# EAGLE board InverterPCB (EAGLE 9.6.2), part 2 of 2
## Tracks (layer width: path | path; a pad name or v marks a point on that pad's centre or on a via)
ADC1_IN8
  Route2 0.25: C57.2 63.3,58.52 | J2.34 65.97,61.19 63.3,58.52 | R124.1 62.62,59.21 63.3,58.52
ADC1_IN10
  Route2 0.25: J2.38 65.44,66.27 C39.2 62.34,63.81 R61.1
ADC1_IN11
  Route15 0.25: J2.36 65.87,66.01 56.33,66.01 C48.2 52.84,69.03 R109.1
ADC2_IN9
  Route2 0.25: J1.24 129.14,48.51 C60.2 122.55,48.51 R129.1
ADC2_IN12
  Route15 0.25: J2.35 71.97,65.01 85.73,65.01 C42.2 88.64,63.3 R99.1
ADC2_IN13
  Route2 0.25: J2.37 73.86,66.27 C51.2 77.61,63.33 R114.1
ADC3_IN0
  Route2 0.25: R104.1 60.71,46.14 63.27,48.7 | J2.28 63.69,49.11 63.27,48.7 | C45.2 63.27,48.7
ADC3_IN1
  Route15 0.25: J2.30 67.05,55.01 54.92,55.01 C54.2 52.53,56.56 R119.1
CURENT_MEAS_DC_LINK
  Top 0.25: IC26.13 IC26.14 | R125.2 230.21,54.75 J23.1
  Route15 0.25: J23.1 232.47,57.01 247.79,57.01 256.15,65.37 IC26.14
CURENT_MEAS_PHASE_1
  Top 0.25: IC26.2 IC26.1
  Top 0.254: IC20.6 250.79,80 250.79,73.01 252.04,71.76 259.04,71.76 260.28,70.52 263.74,70.52 IC26.2
  Bottom 0.254: IC21.7 236.87,84.93 237.79,84.01 246.78,84.01 IC20.6
CURENT_MEAS_PHASE_2
  Top 0.25: IC26.6 IC26.7
  Bottom 0.254: IC26.6 260.84,80.71 259.55,79.42 254.2,79.42 252.29,77.51 IC20.4 245.08,77.51 243.81,78.78 237.02,78.78 235.95,79.85 IC21.5
CURENT_MEAS_PHASE_3
  Top 0.25: IC26.9 IC26.8
  Top 0.254: IC26.8 252.38,87.01 242.46,87.01 IC20.8
  Bottom 0.254: IC20.8 240.58,87.22 239.79,88.01 229.79,88.01 228.79,87.01 228.79,84.01 227.17,82.39 IC21.9
CURRENT_MEAS_PHASE_1_GRID
  Top 0.25: J15.1 253.39,55.17 R105.2
  Bottom 0.2: IC4.1 IC4.2
  Bottom 0.25: R105.2 266.38,61.01 295.51,61.01 IC4.1
CURRENT_MEAS_PHASE_2_GRID
  Top 0.25: J17.1 281.7,55.4 R110.2
  Bottom 0.2: IC4.7 302.66,83.2 302.66,80.76
  Bottom 0.25: J17.1 279.41,60.01 300.79,60.01 304.79,64.01 304.79,79.01 303.04,80.76 302.66,80.76 IC4.6
CURRENT_MEAS_PHASE_3_GRID
  Top 0.25: R115.2 296.79,55.28 J19.1
  Route15 0.25: J19.1 296.74,78.96 296.79,79.01 295.04,80.76 IC4.9 IC4.8
DC_LINK_NEGATIVE_OUT
  Top 0.25: J5.1 85.23,182.66 VR7.1
  Top 1: R36.2 134.95,157.49 D6.A 135.49,166.94 Q2.S | R50.2 D10.A | D10.A | R56.2 274.83,156.03 D13.A 275.34,165.87 Q6.S | Q4.S 204.98,180.14 D10.A
  Bottom 0.25: J5.1 79.93,196.87 79.79,197.01
  Bottom 1: C20.2 123.95,170.01 131.34,170.01 D6.A | C23.2 196.57,172.01 201.79,172.01 204.97,168.83 D10.A | C27.2 265.3,171.01 270.79,171.01 274.83,166.97 D13.A
  Bottom 3: 47.9,187.42 48.5,188.01 55.79,188.01 64.79,197.01 79.79,197.01 128.79,197.01 | 128.79,197.01 135.79,190.01 135.79,180.72 Q2.S | 128.79,197.01 198.79,197.01 | 198.79,197.01 205.79,190.01 205.79,180.95 Q4.S | 198.79,197.01 268.79,197.01 275.34,190.46 275.34,185.01 Q6.S
  Bottom 4: X3.1 19.9,187.42 D2.A | D2.A D3.A 40.27,187.42 | X3.2 14.9,187.42 D2.A | 40.27,187.42 C73.- | C28.2 47.9,187.42 40.27,187.42
DC_LINK_POSITIVE
  Top 0.254: D3.C D2.C 15.74,196.06 X2.2
  Top 4: X2.1 15.8,196.01 | 15.8,196.01 C73.+ 54.13,196.01 C28.1 | X2.2 15.8,196.01
  pour Top: 63.82,183.1 63.82,193.04 57.16,199.7 38.7,199.7 37.74,198.74 37.74,193.05 38.47,192.32 57.53,192.32 57.62,192.41 60.66,189.37 60.66,183.42 60.98,183.1
DC_LINK_POSITIVE_OUT
  Top 0.25: 67.4,187.01 89.34,187.01 R38.2 97.71,185.31 Q1.D
  Top 0.254: 67.4,187.01 66.26,187.01 66.03,186.78 U11.1
  Top 1: Q1.D 103.03,179.99 D4.C | Q3.D 172.79,166.69 D9.C | Q5.D 242.75,165.4 D12.C
  Bottom 1: Q1.D 107.01,176.01 111.54,176.01 R152.1 | Q3.D 177.17,176.01 181.74,176.01 R154.1 | Q5.D 247.31,175.01 250.34,175.01 R155.1
  pour Top: 64.51,184.13 64.48,185.24 64.48,188.13 75.64,199.29 237.2,199.29 244.96,191.53 244.96,176.06 243.86,174.96 241.31,174.96 239.92,176.35 239.92,190.4 236.08,194.24 181.39,194.24 174.82,187.67 174.82,176.86 173.74,175.78 171.64,175.78 170.56,176.86 170.56,187.74 163.81,194.49 108.8,194.57 105.13,190.9 105.13,190.1 105.07,190.04 105.07,176.91 104.65,176.49 100.06,176.49 99.29,177.26 99.29,190.82 95.62,194.49 77.92,194.49 66.33,182.9
DIGITAL_PROTECTION
  Top 0.25: R30.2 R39.1
  Route15 0.25: R39.1 114.87,53.01 122.65,53.01 123.58,52.07 129.59,52.07 129.65,52.01 130.79,52.01 131.7,51.1 J1.25
ENABLE_PWM  (via drill 0.35)
  Top 0.25: T1.3 144.62,58.05 | 144.62,58.05 T12.3 T11.3 160.52,58.05 T10.3 | R85.2 141.79,52.15 141.79,57.01 142.83,58.05 144.62,58.05 | IC22.10 163.95,92.17 165.79,94.01 190.79,94.01 193.43,91.37 IC25.10 | R30.1 v112.79,70.01
  Route2 0.25: IC22.2 156.33,80.55 155.79,80.01 150.79,80.01 144.5,73.72 v144.5,68.01 T1.3
  Route15 0.25: v112.79,70.01 112.79,76.01 113.79,77.01 v120.79,77.01
  Bottom 0.25: IC22.10 163.95,85.01 | 163.95,85.01 IC22.5 | IC22.2 158.98,85.01 163.95,85.01 | IC25.10 193.43,85.01 | 193.43,85.01 IC25.5 | IC25.2 188.26,85.01 193.43,85.01 | v120.79,77.01 135.5,77.01 v144.5,68.01
GPIO_OUTPUT
  Route15 0.254: IC14.15 136.71,43.39 135.47,44.63 130.48,44.63 J1.22
HIGHSIDE_3V  (via drill 0.35)
  Top 0.25: IC17.4 392.44,70.01 400.79,70.01 401.74,69.06 402.51,69.06 C84.1 402.6,68.97 402.6,63.82 401.79,63.01 400.47,63.01 | 400.47,63.01 383.79,63.01 | 383.79,63.01 365.82,63.01 | 365.82,63.01 346.81,63.01 | 346.81,63.01 R40.2 | R26.2 365.82,63.01 | R15.2 381.8,65 383.79,63.01 | R3.2 400.47,63.01 | 346.81,63.01 341.79,63.01 340.76,64.04 C5.1 338.62,69.18 337.79,70.01 329.79,70.01 328.56,68.78 IC19.4 | C85.1 372.76,74 363.19,74 363.18,74.01 362.63,74.01 IC18.11
  Top 1: IC2.2 37.43,152.83 R69.1
  Route15 0.25: R26.2 362.42,66.41 362.42,74.22 IC18.11
  Route15 1: C2.1 76.49,129.01 141.79,129.01 141.79,128.01 142.79,127.01 v144.79,127.01 | v155.79,127.01 157.79,129.01 213.79,129.01 v215.79,127.01 | v226.79,127.01 228.79,129.01 283.79,129.01 v285.79,127.01 | v303.79,127.01 305.79,129.01 328.79,129.01 338.79,119.01 338.79,71.16 C5.1
  Bottom 0.25: VR1.3 328.56,60.87 IC19.4
  Bottom 1: C2.1 50.12,155.38 50.12,155.89 48.1,157.91 R69.1 | v144.79,127.01 v155.79,127.01 | v215.79,127.01 v226.79,127.01 | v285.79,127.01 v303.79,127.01
HIGHSIDE_5V
  Top 1: C83.1 43.78,141.4 IC5.3 | OK1.8 103.61,128.6 R43.1 96.12,136.09 R42.1 96.16,137.52 C11.1 | C19.1 R52.1 164.94,135.45 R53.1 172.61,127.79 OK2.8 | C24.1 234.64,139.6 R58.1 237.18,132.12 R59.1 242.27,125.76 OK3.8
  Bottom 1: C83.1 93.46,140.13 R42.1 97.58,136.01 164.79,136.01 164.94,136.16 R52.1 167.15,134.66 R58.1
HIGHSIDE_15V_VB  (via drill 0.35)
  Top 1: C15.1 106.28,148.74 U4.8 | D5.C 127.99,146.01 v111.79,146.01
  Bottom 1: v111.79,146.01 108.88,146.01 U4.8
HIGHSIDE_15V_VB1  (via drill 0.35)
  Top 1: C13.1 36.19,127.4 IC9.3 | U4.5 114.92,147.58 C14.1 120.75,147.58 R153.1 | R156.1 189.53,146.73 C21.1 183.91,146.73 U6.5 | R157.1 259.03,144.76 C25.1 253.62,144.76 U7.5
  Route2 1: C13.1 54.56,137.01 v84.79,137.01
  Route15 1: v84.79,137.01 91.79,144.01 112.79,144.01 116.36,147.58 C14.1
  Bottom 1: R153.1 134.56,149.78 139.79,155.01 180.79,155.01 182.8,153 U6.5 | R156.1 195.98,149.2 198.79,152.01 250.79,152.01 252.43,150.37 U7.5
HIGHSIDE_-3V  (via drill 0.35)
  Top 0.25: C84.2 401.9,74.12 400.79,73.01 392.45,73.01 IC17.11 | C85.2 370.58,69.22 369.79,70.01 363.06,70.01 IC18.4
  Top 1: IC3.3 38.7,171.88 R67.2 52.67,171.88 C3.2
  Route2 0.25: C5.2 339.51,73.01 v332.79,73.01
  Route15 0.2: 361.04,68.76 IC18.4
  Route15 0.25: C5.2 350.54,74.26 354.79,70.01 359.79,70.01 360.93,68.88 361.04,68.76 | v332.79,73.01 331.29,73.01 IC19.11
  Route15 1: C3.2 60.79,163.76 60.79,151.01 80.79,131.01 v144.79,131.01 | v157.79,131.01 v215.79,131.01
  Bottom 0.25: C85.2 375.25,71.41 388.19,71.41 390.14,73.36 IC17.11
  Bottom 1: v144.79,131.01 v157.79,131.01 | C5.2 340.76,119.04 327.04,132.76 235.54,132.76 233.79,131.01 v215.79,131.01
HIGHSIDE_GND  (via drill 0.35)
  Top 1: X1.2 15.12,168.59 D1.A 25.48,168.59 C4.2 30.53,168.07 31.8,166.8 IC3.2 | C82.2 28.54,138.86 IC5.2 41.24,138.86 C83.2 | C12.2 29.84,127.46 32.41,124.89 IC9.2 42.38,124.89 C13.2 | C14.2 117.63,143.37 112.95,143.37 111.29,141.72 U4.3 111.29,141.67 108.95,144.01 99,144.01 C11.2 | C21.2 186.43,142.43 181.93,142.43 180.26,140.76 U6.3 180.26,140.78 178.03,143.01 168.79,143.01 C19.2 | C24.2 238.82,140.53 248.28,140.53 249.89,138.93 U7.3 249.89,138.87 251.61,140.59 255.96,140.59 C25.2
  Route2 1: v342.79,88.29 327.07,88.29 323.48,84.7 IC19.13 IC19.12
  Bottom 1: C4.2 29.59,164.48 29.59,144.99 C82.2 | C13.2 49.19,126.56 49.19,131.91 46.05,135.05 C83.2 41.79,138.31 41.79,142.01 43.79,144.01 93.32,144.01 C11.2 | C14.2 120.28,142.5 121.79,144.01 162.1,144.01 C19.2 | C21.2 189.96,141.65 192.39,144.08 234.05,144.08 C24.2 | C25.2 259.37,142.19 320.84,142.19 342.79,120.24 v342.79,88.29
HIGHSIDE_LOW_VOLTAGE_INPUT
  Top 1: X1.1 19.09,161.76 D1.C 24.09,156.77 C1.1 27.3,155.37 IC2.3 | C82.1 IC5.1 | C12.1 36.13,122.38 IC9.1
  Bottom 1: IC2.3 36.14,155.35 32.91,155.35 31.89,154.33 31.89,137.43 33,136.32 | IC5.1 33,136.32 | 33,136.32 31.91,135.23 31.91,124.04 33.63,122.32 36.13,122.32 IC9.1
HIGHSIDE_SPLIT_GND  (via drill 0.35)
  Top 0.2: U1.4 391.97,50.89 378.03,50.89 376.35,52.57
  Top 0.25: U1.4 393.64,58.86 396.79,62.01 403.79,62.01 404.79,63.01 404.79,75.01 402.79,77.01 394.36,77.01 IC17.10 | v371.79,61.01 376.35,56.45 U2.4 376.35,52.57 374.79,51.01 360.44,51.01 | U3.4 360.44,51.01 | 360.44,51.01 341.72,51.01 U5.4 340.11,52.69 336.79,56.01 336.79,63.01 334.79,65.01 327.79,65.01 326.02,66.79 IC19.3 | R12.2 397,154.01 388.62,154.01 R17.2
  Top 1: VR3.2 51.4,166.8 53.94,164.26 C3.1 C2.2 51.4,155.37 | 51.4,155.37 VR2.2 | C4.1 29.01,162.99 32.19,159.81 46.96,159.81 51.4,155.37
  Route2 0.25: v371.79,61.01 370.55,61.01 IC18.5 | v381.79,88.01 381.79,84.01 386.79,79.01 388.99,79.01 IC17.10
  Route2 1: C2.2 71.43,155.37 97.79,129.01 v144.79,129.01 114.54,129.01 OK1.5 | IC19.10 331.1,73.2 IC19.3
  Bottom 0.25: R17.2 383.79,153.15 383.79,118.01 | R28.2 372.75,121.05 374.79,119.01 382.79,119.01 383.79,118.01 | 383.79,118.01 383.79,99.01 381.79,97.01 v381.79,88.01
  Bottom 1: C4.1 23.19,160.18 23.19,154.4 C1.2 | v144.79,129.01 181.79,129.01 | 181.79,129.01 251.79,129.01 | OK2.5 180.23,127.45 181.79,129.01 | OK3.5 249.89,127.11 251.79,129.01 | IC19.10 331.1,78.31 331.79,79.01 335.79,79.01 338.79,82.01 338.79,117.43 327.21,129.01 251.79,129.01
HIGHSIDE_VOFFSET  (via drill 0.35)
  Top 0.2: 358.5,70.58 375.75,70.58 v375.77,70.6
  Top 0.25: C18.1 330.65,56.74 VR1.2 320.47,56.74 J3.2 | IC18.3 358.5,70.58 IC18.12
  Bottom 0.2: IC17.5 392.68,68.73 390.81,70.6 v375.77,70.6
  Bottom 0.25: C18.1 349.77,59.25 IC18.3
LACH_RESET  (via drill 0.35)
  Top 0.25: R81.2 153.59,24.09 SW1.P$2 | IC14.6 173.51,52.25 168.43,52.25 IC14.12 169.76,48.44 | IC14.4 171.07,48.47 171.03,48.44 169.76,48.44 | IC14.14 169.7,48.44 169.76,48.44
  Route2 0.25: R81.2 155.89,24.11 158.79,27.01 v158.79,34.01
  Route15 0.25: v158.79,34.01 161.79,37.01 168.79,37.01 170.79,39.01 170.79,44.01 168.87,45.93 IC14.14
LOWSIDE_3.3V  (via drill 0.35)
  Top 0.25: IC16.4 215.79,24.75 215.79,32.25 C7.1 | IC26.4 263.68,75.63 261.79,77.51 261.79,86.62 C87.1 | C6.1 322.04,34.96 322.04,27.1 324.34,24.8 IC7.4 | IC1.4 214.79,44.44 v214.79,44.01 | v225.79,61.01 258.79,61.01 | v312.79,42.01 310.79,44.01 310.79,69.01 304.12,75.68 IC4.4 | C29.2 295.96,170.62 U10.8 | C74.2 330.35,170.52 U12.8 | C75.2 344.58,134.71 U13.8 | C76.2 359.15,100.37 U14.8 | C10.2 223.76,170.49 U9.8 | C8.2 152.75,171.18 U8.8 | U11.8 66.03,176.25 C33.2 65.79,174.5 65.79,97.93 C32.1
  Top 0.254: 258.79,61.01 263.79,61.01 266.79,64.01 266.79,74.01 265.18,75.62 263.78,75.62 IC26.4
  Top 1: IC15.2 39.97,93.7 R64.1 56.48,88.62 C32.1
  Route2 1: C32.1 72.87,105.01 v153.79,105.01
  Route15 0.25: v214.79,44.01 214.79,35.98 C7.1 | C86.1 221.11,60.34 221.79,61.01 v225.79,61.01 | C6.1 314.99,42.01 v312.79,42.01 | C87.1 262.47,99.33 256.79,105.01 | C8.2 153.24,105.56 v153.79,105.01 | C10.2 224.26,114.54 233.79,105.01 | 285.56,102.78 296.54,113.75 C29.2 300.56,166.01 327.79,166.01 330.74,168.96 C74.2 330.74,137.06 336.79,131.01 341.9,131.01 C75.2 345.09,105.71 352.79,98.01 357.69,98.01 C76.2
  Route15 1: v153.79,105.01 233.79,105.01 256.79,105.01 283.33,105.01 285.56,102.78 C88.1
  Bottom 0.25: C88.1 299.81,86.41 299.81,78.03 302.16,75.68 IC4.4 | C86.1 215.79,58.48 215.79,51.59 IC1.4
LOWSIDE_5V
  Top 0.2: C37.1 170.97,60.03 C34.1
  Top 0.25: R85.1 149.51,34.27 R81.1 155.31,36.01 166.46,36.01 | 202.06,36.01 R127.1 | 166.46,36.01 167.22,36.01 | 167.22,36.01 177.79,36.01 | 177.79,36.01 180.05,36.01 | 180.05,36.01 190.79,36.01 | 202.06,36.01 190.79,36.01 | R142.1 190.79,34.48 190.79,36.01 | R128.1 177.94,35.86 177.79,36.01 | R66.1 166.44,35.99 166.46,36.01 | IC14.16 167.19,36.04 167.22,36.01 | IC11.14 180,36.06 180.05,36.01 | R112.1 205.05,40.01 | 205.05,40.01 205.05,39 202.06,36.01 | 205.05,40.01 205.15,40.11 R113.1 205.05,44.49 R117.1 205.05,52.56 R149.1 204.96,52.65 R151.1 204.95,56.45 204.95,60.16 204.93,60.17 R150.1 204.97,62.43 206.09,63.55 225.33,63.55 226.79,65.01 231.74,65.01 C71.1 235.64,66.01 244.48,66.01 C69.1 | C91.1 202.44,88.01 183.79,88.01 | 183.79,88.01 183.27,88.53 IC25.14 181.84,88.75 C70.1 172.85,88.01 154.79,88.01 | 154.79,88.01 153.79,89.01 153.79,89.9 | VR10.3 154.07,75.73 151.79,78.01 151.79,85.01 154.79,88.01 | VR11.3 182.07,75.73 181.79,76.01 181.79,86.01 183.79,88.01 | 136.78,107 136.76,107.01 103.79,107.01 | C89.1 64.5,25.63 J2.6
  Top 1: IC10.3 49.33,81 C17.1 60.63,81.07 R130.1 96.48,113.88 R131.1 103.35,107.01 103.79,107.01 103.81,107 136.78,107 IC22.14 153.79,89.9 | R135.1 235.39,112.8 R134.1 225.26,106.01 173.59,106.01 R133.1 165.56,114.04 R68.1
  Route2 0.25: C37.1 166.12,62.68 159.79,69.01 159.79,72.68 VR10.3
  Bottom 0.25: IC14.5 170.79,55.03 170.79,60.22 C37.1 | C34.1 177.38,56.22 177.38,43.36 179.86,40.88 IC11.14 | R133.1 173.59,106.01 C70.1 | C89.1 48.38,24.42 42.79,30.01 42.79,74.46 C17.1 | C71.1 233.19,73.51 IC21.3 | C69.1 246.88,73.65 IC20.3
LOWSIDE_GND  (via drill 0.35)
  Top 0.2: U10.6 293.42,172 292.15,170.73
  Top 0.25: T10.1 155.41,55.43 T11.1 T12.1 144.62,55.51 T1.1 | SW1.P$1 156.79,15.59 156.79,19.01 157.95,20.17 T2.1 163.36,20.23 T9.1 186.99,20.23 T8.1 199.79,20.26 T7.1 201.82,22.25 IC16.11 213.32,24.91 213.32,32.36 C7.2 208.79,36.9 208.79,50.01 | C86.2 208.79,56.56 208.79,50.01 | 208.79,50.01 210.29,48.51 IC1.11 | VR10.1 170.8,75.73 C35.2 173.64,83.62 | 173.64,83.62 C70.2 | 173.64,83.62 172.38,82.36 IC22.7 164.38,87.01 v161.79,87.01 | VR11.1 201.11,75.73 C36.2 C91.2 202.07,82.56 IC25.7 194.06,87.01 v189.79,87.01 | IC22.13 IC22.12 | IC25.13 IC25.12 | IC21.12 IC21.11 IC21.10 | IC26.11 257.41,75.63 258.79,77.01 258.79,85.9 C87.2 259.1,89.01 269.3,89.01 270.79,87.52 | C72.2 270.79,87.52 | 270.79,87.52 277.64,87.52 C30.2 284.11,87.49 C79.2 290.46,87.45 290.49,87.47 | 290.49,87.47 C81.2 | C80.2 283.87,70.82 C78.2 290.72,70.76 C77.2 294.81,70.73 IC4.13 | C88.2 290.49,87.47 | U5.5 340.15,44.96 J12.2 | U3.5 358.85,40.35 J10.2 | U2.5 376.39,44.95 J8.2 | U1.5 J4.2 | C89.2 64.62,28.17 J2.8 | C29.1 292.15,170.73 U10.5 | C74.1 326.54,171.02 U12.5 U12.6 | C75.1 340.77,134.97 U13.5 U13.6 | C76.1 355.34,100.75 U14.5 U14.6 | C10.1 219.95,170.76 U9.5 U9.6 | C8.1 148.94,171.47 U8.5 U8.6 | 62.22,180.01 62.22,176.01 C33.1 62.3,175.5 63.79,174.01 63.79,101.01 C32.2 | 62.22,180.01 U11.5 | U11.6 62.81,180.01 62.22,180.01
  Top 0.254: IC20.12 IC20.11
  Top 1: X4.2 15.12,99.3 D7.A 26.75,99.3 C31.2 | C16.2 30.91,78.46 IC10.2 46.93,78.46 C17.2 | VR8.2 56.48,93.7 C32.2 | v159.79,103.01 v231.79,103.01
  Route2 0.25: IC22.12 159.79,90.9 v159.79,103.01 148.16,114.64 C8.1 | 233.79,103.01 233.79,94.01 232.79,93.01 | 232.79,93.01 230.79,91.01 230.79,80.01 228.09,77.31 IC21.11 | IC20.10 239.75,80.05 238.79,81.01 238.79,87.01 232.79,93.01 | C10.1 219.18,115.62 v231.79,103.01 | C29.1 291.46,170.01 | 291.46,170.01 291.46,115.68 278.79,103.01 | 291.46,170.01 295.46,166.01 321.53,166.01 C74.1 325.66,138.14 330.79,133.01 338.82,133.01 C75.1 340.01,114.44 C76.1
  Route2 1: C17.2 51.42,78.01 67.79,78.01 92.79,103.01 v159.79,103.01 | v231.79,103.01 233.79,103.01 278.79,103.01 280.25,103.01 C88.2
  Route15 1: VR8.2 49.48,93.7 47.21,91.43 47.21,78.18 C17.2
  Bottom 0.25: C45.1 63.27,34.5 | 63.27,34.5 63.27,29.52 C89.2 48.3,29.5 45.79,32.01 45.79,55.01 | 64.79,49.9 C57.1 53.46,51.39 C54.1 53.38,52.42 51.79,54.01 46.79,54.01 45.79,55.01 | 64.79,49.9 64.79,36.01 63.27,34.5 | 64.79,67.08 C39.1 60.67,68.89 55.73,63.95 C48.1 53.31,65.49 51.79,67.01 46.79,67.01 45.79,68.01 | 64.79,67.08 64.79,49.9 | 72.2,73.01 C51.1 87.41,68.41 C42.1 | 72.2,73.01 67.79,73.01 64.79,70.01 64.79,67.08 | 72.2,73.01 117.79,73.01 117.79,49.34 C60.1 | C37.2 174.81,61.28 IC14.8 | 183.62,62.68 C34.2 187.62,58.69 IC11.7 185.9,56.12 183.79,54.01 183.79,49.75 | 183.62,62.68 C37.2 | C37.2 173.4,63.29 J6.1 | J7.1 191.53,62.68 183.62,62.68 | C86.2 209.34,63.56 | J7.1 198.06,64.84 199.34,63.56 209.34,63.56 | IC11.12 183.79,49.75 | IC11.13 183.79,47.21 183.79,49.75 | VR10.1 167.92,68.85 J6.1 | J7.1 198.06,75.7 VR11.1 | IC25.12 191.52,87.01 v189.79,87.01 | IC22.12 158.87,89.93 v161.79,87.01 | IC4.13 IC4.12 IC4.11 295.44,75.68 297.78,78.03 297.78,85.48 C88.2 | C44.1 260.3,20.5 262.79,18.01 | C53.1 301.72,39.08 | 301.72,39.08 301.65,39.01 284.4,39.01 | C50.1 284.4,39.01 | 284.4,39.01 262.67,39.01 | 262.67,39.01 C47.1 | 262.67,39.01 246.79,39.01 | 246.79,39.01 244.79,39.01 | 244.79,39.01 238.7,39.01 C59.1 | C38.1 301.53,18.01 | C41.1 284.5,18.01 | 301.53,18.01 284.5,18.01 | 284.5,18.01 262.79,18.01 | 262.79,18.01 248.79,18.01 | 248.79,18.01 238.65,18.01 C56.1 | C71.2 230.66,61.01 239.2,61.01 | 239.2,61.01 C69.2 241.8,73.75 IC20.12 | 239.2,61.01 242.79,61.01 244.79,59.01 244.79,56.01 | 244.79,56.01 244.79,41.01 246.79,39.01 | IC26.11 249.79,69.27 249.79,61.01 244.79,56.01 | C71.2 209.34,63.56 | 301.72,39.08 323,39.08 | 323,39.08 C6.2 324.79,35.16 324.79,33.01
  Bottom 0.25: 323,39.08 338.98,39.08 J12.2 358.88,40.25 J10.2 376.37,40.28 J8.2 393.55,40.3 J4.2 | 324.79,32.21 324.76,32.23 324.76,27.88 | 324.79,32.21 IC7.6 | 324.79,33.01 324.79,32.21 | 324.76,27.88 324.76,24.99 | 324.76,24.99 324.76,24.61 IC7.3 | 324.76,27.88 321.68,24.8 IC7.11 | 324.79,33.01 321.66,29.88 IC7.9 | 324.76,24.99 IC7.13 317.78,18.01 301.53,18.01 | 248.79,18.01 246.79,20.01 246.79,37.01 244.79,39.01 | J6.1 165.08,66.01 141.79,66.01 134.79,73.01 | 45.79,68.01 45.79,72.38 C17.2 | 45.79,55.01 45.79,68.01 | C71.2 228.11,73.49 IC21.12 | T10.1 163.21,55.43 163.79,56.01 163.79,64.72 J6.1 | T1.1 140.79,51.92 140.79,22.01 135.79,17.01 125.79,17.01 123.7,19.1 C60.1 | R39.2 112.79,40.01 115.79,37.01 119.79,37.01 123.7,40.92 C60.1
  Bottom 0.3: 117.79,73.01 134.79,73.01
  Bottom 1: C16.2 33.09,85.78 33.09,93.01 28.59,97.51 C31.2
N$1  (via drill 0.35)
  Top 0.25: U1.1 401.26,57.48 401.79,58.01 405.79,58.01 408.79,61.01 408.79,77.01 404.79,81.01 v398.79,81.01
  Route2 0.25: v398.79,81.01 398.79,76.36 IC17.8
N$2
  Top 0.25: R3.1 398.75,52.59 U1.2
N$3  (via drill 0.35)
  Top 0.25: R13.2 403.82,131.56 R1.1 398.9,123.9 400.12,122.68 400.12,110.68 400.79,110.01 v400.79,100.01
  Route2 0.25: v400.79,100.01 400.79,67.01 399.79,66.01 386.75,66.01 IC17.2
N$4  (via drill 0.35)
  Top 0.25: U1.3 396.18,54.49 R11.1 396.09,59.31 396.79,60.01 404.79,60.01 406.79,62.01 406.79,76.01 403.79,79.01 v395.79,79.01
  Route2 0.25: v395.79,79.01 395.79,75.9 IC17.9
N$5
  Top 0.25: R4.2 386.38,126.39 VR4.2
N$6  (via drill 0.35)
  Top 0.25: R11.2 385.48,64.73 IC17.1
  Route15 0.25: v383.79,85.01 383.79,68.98 IC17.1
  Bottom 0.25: VR4.3 385.69,98.91 383.79,97.01 v383.79,85.01
N$7  (via drill 0.35)
  Top 0.25: R2.1 398.84,121.46 R1.2 398.9,109.9 399.79,109.01 v399.79,100.01
  Route2 0.25: v399.79,100.01 399.79,69.74 IC17.7
N$8
  Top 0.25: R10.2 R12.1
  Bottom 0.25: R12.1 401.79,163.44 401.79,102.01 404.79,99.01 404.79,68.01 402.79,66.01 389.29,66.01 IC17.3
N$9  (via drill 0.35)
  Top 0.25: R2.2 391.39,131.62 R4.1 | v400.79,128.01 400.79,112.01 401.79,111.01 v401.79,100.01
  Route2 0.25: R4.1 393.91,129.01 399.79,129.01 v400.79,128.01 | v401.79,100.01 v401.79,76.01
  Route15 0.25: v401.79,76.01 395.22,69.44 IC17.6
N$10
  Top 0.25: R5.2 406.5,156.04 R10.1
N$11
  Top 0.25: R6.2 406.55,121.44 R13.1
N$12  (via drill 0.35)
  Top 0.25: U2.1 383.97,54.83 v376.79,62.01
  Route2 0.25: v376.79,62.01 370.82,67.98 IC18.7
N$13
  Top 0.25: R15.1 381.45,52.63 U2.2
N$14  (via drill 0.35)
  Top 0.25: U2.3 378.87,52.63 R16.1 378.87,56.93 v374.79,61.01
  Route2 0.25: v374.79,61.01 369.79,66.01 368.09,66.01 IC18.6
N$15
  Top 0.25: R16.2 378.87,74.09 380.1,75.32 IC17.14 382.52,85.19 VR5.3
N$16  (via drill 0.35)
  Top 0.25: R9.2 391.74,166.15 R17.1
  Route15 0.25: v387.79,85.01 387.79,75.52 IC17.12
  Bottom 0.25: R17.1 386.63,162.17 387.79,161.01 v387.79,85.01
N$17
  Top 0.25: R18.2 398.47,95.93 R7.1 398.46,93.68 392.79,88.01 392.79,85.01 385.06,77.28 IC17.13
N$18
  Top 0.25: R7.2 395.65,85.76 R8.1
  Bottom 0.25: R8.1 393.9,84.01 384.79,84.01 381.79,81.01 381.79,78.01 376.08,72.3 357.74,72.3 IC18.1
N$19
  Top 0.25: R8.2 391.03,95.85 R20.1 385.55,95.77 382.79,93.01 382.79,87.01 381.79,86.01 381.79,78.01 377.79,74.01 377.79,69.01 374.79,66.01 357.93,66.01 IC18.2
N$20
  Top 0.25: R20.2 385.94,90.62 VR5.2
N$21
  Top 0.25: R21.2 394.43,156.04 R9.1
N$22
  Top 0.25: R22.2 403.48,85.75 R18.1
N$23  (via drill 0.35)
  Top 0.25: v364.79,49.01 339.79,49.01 334.79,54.01 334.79,61.01 332.79,63.01 323.79,63.01 320.94,65.87 IC19.1
  Route2 0.25: U3.1 366.47,49.69 365.79,49.01 v364.79,49.01
N$24
  Top 0.25: R26.1 U3.2
N$25  (via drill 0.35)
  Top 0.25: R27.1 361.41,52.62 U3.3 | v360.79,50.01 340.79,50.01 335.79,55.01 335.79,62.01 333.79,64.01 324.79,64.01 323.48,65.33 IC19.2
  Route2 0.25: U3.3 361.39,50.61 v360.79,50.01
N$26
  Top 0.25: VR6.3 368.66,78.32 IC18.8
  Route2 0.25: R27.2 362.42,65.92 362.42,70.53 362.9,71.01 366.79,71.01 368.66,72.88 IC18.8
N$27
  Top 0.25: R25.2 372.17,131.17 R28.1
  Bottom 0.25: R28.1 370.79,129.87 370.79,120.01 372.79,118.01 381.79,118.01 382.79,117.01 382.79,100.01 380.79,98.01 380.79,78.01 375.87,73.09 364.71,73.09 363.58,74.22 IC18.10
N$28  (via drill 0.35)
  Top 0.25: R29.2 371.78,95.94 R23.1 371.79,95.93 371.79,90.01 372.79,89.01 372.79,85.01 v368.79,81.01
  Route2 0.25: v368.79,81.01 366.12,78.34 IC18.9
N$29  (via drill 0.35)
  Top 0.25: R23.2 369.17,85.83 R24.1 366.79,83.45 v366.79,83.01 | v364.33,80.57 363.77,80.01 355.79,80.01 353.42,77.64 IC18.14
  Route2 0.25: v366.79,83.01 364.35,80.57 v364.33,80.57
N$30  (via drill 0.35)
  Top 0.25: R24.2 364.08,95.97 R31.1 364.06,88.74 365.79,87.01 365.79,85.01 v364.79,84.01 | v361.79,79.35 358.13,79.35 355.96,77.18 IC18.13
  Route2 0.25: v364.79,84.01 364.79,82.35 v361.79,79.35
N$31
  Top 0.25: R31.2 358.83,91.05 VR6.2
N$32
  Top 0.25: R32.2 377.19,121.06 R25.1
N$33
  Top 0.25: R33.2 376.65,85.84 R29.1
N$34
  Route2 0.25: T1.2 147.79,55.52 147.79,50.11 R60.1
N$35
  Top 1: IC15.1 42.51,96.24 R64.2 47.59,96.24 VR8.1
N$36
  Top 1: D5.A 124.6,141.28 R153.2
N$37
  Top 1: X4.1 15.12,90.65 D7.C 26.75,90.65 C31.1 29.81,91.16 IC15.3 | C16.1 39.94,75.95 IC10.1
  Bottom 1: IC15.3 35.79,88.25 35.79,78.01 37.88,75.92 IC10.1
N$38  (via drill 0.35)
  Top 0.25: J5.2 79.96,180.09 VR7.2 86.1,180.09 R38.1 91.04,125.76 94.79,122.01 327.79,122.01 333.79,116.01 v333.79,82.01
  Route15 0.25: v333.79,82.01 334.79,81.01 334.79,69.28 IC19.6
N$39
  Top 0.25: R40.1 345.12,52.7 U5.2
N$40
  Top 1: R34.1 97.1,164.67 | 97.1,164.67 Q1.G | R37.1 97.1,158.4 97.1,164.67
N$41
  Top 1: U4.1 106.21,137.54 | 106.21,137.54 R42.2 | OK1.7 106.15,137.48 106.21,137.54
N$42
  Top 1: R35.1 124.49,164.46 | 124.49,164.46 Q2.G | R36.1 124.49,157.79 124.49,164.46
N$43  (via drill 0.35)
  Top 0.25: U1.6 403.41,37.71 R44.2 399.41,30.01 339.79,30.01 v333.79,24.01
  Route2 0.25: v333.79,24.01 329.5,19.72 IC7.2
N$44
  Top 1: U4.2 108.75,133.62 | 108.75,133.62 R43.2 | OK1.6 108.69,133.56 108.75,133.62
N$45  (via drill 0.35)
  Top 1: v117.79,150.01 120.33,152.55 R35.2
  Bottom 1: U4.4 113.83,146.05 v117.79,150.01
N$46
  Top 1: R34.2 101.08,147.01 107.79,147.01 108.75,147.97 U4.7
N$47  (via drill 0.35)
  Top 0.25: U5.1 347.73,60.95 v347.79,61.01 | v346.79,66.01 342.79,70.01 342.79,75.01 342.06,75.74 IC19.8
  Route2 0.25: v347.79,61.01 347.79,65.01 v346.79,66.01
N$48  (via drill 0.35)
  Top 0.25: U5.3 342.65,54.37 R41.1 340.31,54.49 337.79,57.01 337.79,64.01 v335.79,66.01
  Bottom 0.25: v335.79,66.01 334.79,67.01 334.79,74.59 IC19.9
N$49  (via drill 0.35)
  Top 1: U6.8 175.18,150.89 C22.1 | D8.C 195.28,144.57 v180.42,144.57
  Bottom 1: v180.42,144.57 178.45,144.57 U6.8
N$50
  Top 0.25: U2.6 386.12,37.76 R45.2 383.97,32.01 335.71,32.01 331.04,27.34 IC7.5
N$51
  Route2 0.25: R60.2 150.73,37.01 172.79,37.01 174.81,39.03 IC14.1
  Bottom 0.25: R65.2 160.6,37.01 150.73,37.01 R60.2
N$52  (via drill 0.35)
  Top 0.25: U8.7 151.48,123.31 v151.79,123.01
  Route2 0.25: v238.79,100.01 264.79,100.01 273.79,91.01 273.79,86.01 277.39,82.41 C30.1
  Route15 0.25: v154.79,100.01 v238.79,100.01
  Bottom 0.25: v151.79,123.01 151.79,103.01 v154.79,100.01
  Bottom 0.254: IC26.3 266.87,73.09 273.79,80.01 276.19,82.41 C30.1
N$53  (via drill 0.35)
  Top 1: C26.1 U7.8 | D11.C 265.03,142.64 250.05,142.64 v250.03,142.62
  Bottom 1: v250.03,142.62 248.14,142.62 U7.8
N$54
  Route2 0.25: R41.2 339.06,68.12 IC19.7 334.06,66.01 333.21,66.01 IC19.5
N$55  (via drill 0.35)
  Top 0.25: IC26.5 266.49,78.17 C72.1 | U9.7 222.5,124.31 v222.79,124.01
  Bottom 0.25: v222.79,124.01 222.79,114.16 250.79,86.16
  Bottom 0.254: 250.79,86.16 251.94,85.01 268.19,85.01 C72.1
N$56  (via drill 0.35)
  Top 0.25: U3.6 368.71,37.66 R46.2 367.86,33.01 333.66,33.01 329.15,28.5 v323.43,28.5
  Route2 0.25: v323.43,28.5 322.28,27.34 IC7.10
N$57
  Top 1: IC3.1 38.7,161.72 R67.1 42.51,162.99 VR3.3
N$58
  Top 1: VR2.1 45.05,150.29 R69.2 39.97,150.29 IC2.1
N$59  (via drill 0.35)
  Top 0.25: C77.1 292.09,74.47 301.23,74.47 IC4.3 | U12.7 328.79,174.47 328.79,163.01 326.79,161.01 301.79,161.01 298.79,158.01 v298.79,124.01
  Route2 0.25: v298.79,124.01 298.79,76.91 IC4.3
N$60  (via drill 0.35)
  Top 0.25: U5.6 350,37.66 R47.2 352.59,36.01 336.79,36.01 334.79,38.01 318.79,38.01 v317.79,37.01
  Route2 0.25: v317.79,37.01 312.79,32.01 312.79,26.01 316.54,22.26 IC7.12
N$61
  Bottom 0.25: T2.2 161.4,22.17 R65.1
N$63  (via drill 0.35)
  Top 0.25: v282.79,78.01 287.18,82.4 C81.1 | U11.7 v64.76,104.04
  Route2 0.25: IC26.12 258.87,73.09 259.87,74.09 270.87,74.09 274.79,78.01 v282.79,78.01
  Route15 0.25: IC26.12 254.71,73.09 251.79,76.01 251.79,90.01 240.79,101.01 67.79,101.01 v64.76,104.04
N$64
  Bottom 0.25: LED2.A 166.44,21.12 R66.2
N$65
  Top 1: R48.1 167.29,164.29 | 167.29,164.29 Q3.G | R51.1 167.29,158.23 167.29,164.29
N$66
  Top 1: R50.1 194.3,158.08 194.3,164.05 | 194.3,164.05 Q4.G | R49.1 194.3,164.05
N$67
  Top 1: U6.1 175.18,136.94 175.15,136.91 | 175.15,136.91 R52.2 | OK2.7 175.15,136.91
N$68
  Top 1: U6.2 177.72,132.85 | 177.72,132.85 R53.2 | 177.72,132.85 177.72,125.65 OK2.6
N$69
  Top 1: R48.2 171.76,146.01 175.89,146.01 U6.7
N$70  (via drill 0.35)
  Top 1: v186.79,149.01 189.62,151.84 R49.2
  Bottom 1: U6.4 182.8,145.02 v186.79,149.01
N$71
  Top 1: D8.A 194.57,141.61 R156.2
N$74
  Top 1: R54.1 237.25,162.07 | 237.25,162.07 Q5.G | R57.1 237.25,155.65 237.25,162.07
N$75
  Top 1: R55.1 264.34,162.79 | 264.34,162.79 Q6.G | R56.1 264.34,156.36 264.34,162.79
N$76
  Top 1: U7.1 R58.2 OK3.7
N$77
  Top 1: U7.2 247.34,138.33 R59.2 247.34,125.18 OK3.6
N$78
  Top 1: R54.2 243.03,142.53 246.31,142.53 247.35,143.57 U7.7
N$79  (via drill 0.35)
  Top 1: v255.98,146.52 260.34,150.88 R55.2
  Bottom 1: U7.4 252.43,142.97 v255.98,146.52
N$80
  Top 1: D11.A 264.18,139.75 R157.2
N$84  (via drill 0.35)
  Top 0.25: R19.1 309.04,24.14 C38.2 305.61,17.01 249.79,17.01 v248.79,16.01
  Route15 0.25: v248.79,16.01 244.79,16.01 243.79,17.01 220.99,17.01 IC16.3
N$86
  Top 0.25: C61.1 299.78,25.43 C9.1 300.95,24.25 R14.1 309.08,28.72 R19.2
N$87  (via drill 0.35)
  Top 0.25: C78.1 286.19,75.84 287.37,77.01 301.35,77.01 IC4.5 | U13.7 343.31,130.53 v332.79,120.01
  Route2 0.25: v332.79,120.01 306.79,94.01 306.79,82.45 IC4.5
N$88  (via drill 0.35)
  Top 0.25: C41.2 287.18,20.41 R63.1
  Route2 0.25: C41.2 287.24,17.46 285.79,16.01 262.79,16.01 261.79,15.01 v250.79,15.01
  Bottom 0.25: v250.79,15.01 228.07,15.01 IC16.5
N$89
  Top 0.25: T2.3 164.69,17.63 LED2.K
N$90
  Top 0.25: C40.1 278.32,25.32 C62.1 279.67,24.11 R62.1 287.18,28.71 R63.2
N$91
  Top 0.25: IC14.3 175.89,47.01 186.57,47.01 IC11.3
N$93  (via drill 0.35)
  Top 0.25: v276.95,79.42 279.89,82.37 C79.1 | U10.7 294.69,124.12 v294.79,124.01
  Route2 0.25: IC26.10 258.95,78.17 260.2,79.42 v276.95,79.42
  Bottom 0.25: v294.79,124.01 294.79,98.01 285.79,89.01 285.79,83.01 285.15,82.37 C79.1
N$94  (via drill 0.35)
  Top 0.25: C44.2 265.34,20.7 R101.1 | v260.79,16.01 250.79,16.01 249.79,15.01 221.79,15.01 217.79,11.01 210.79,11.01 207.79,14.01 v207.79,21.01
  Route2 0.25: v207.79,21.01 207.79,21.91 IC16.10
  Route15 0.25: C44.2 260.79,16.07 v260.79,16.01
N$95
  Top 0.25: C43.1 256.43,25.38 C63.1 257.5,24.36 260.79,24.36 | 260.79,24.36 R100.1 | R101.2 265.34,28.91 260.79,24.36
N$96  (via drill 0.35)
  Top 0.25: C80.1 281.62,75.9 281.65,75.87 282.54,75.87 284.9,78.22 IC4.10 296.27,79.55 306.33,79.55 v306.79,80.01 | U14.7 357.79,104.28 357.79,100.01 355.79,98.01 v335.79,98.01
  Route15 0.25: v335.79,98.01 312.79,98.01 307.79,93.01 307.79,81.01 v306.79,80.01
N$99  (via drill 0.35)
  Top 0.25: C47.2 265.46,41.3 R106.1 267.79,47.3 267.79,55.01 263.79,59.01 v220.79,59.01
  Route2 0.25: v220.79,59.01 219.79,58.01 214.79,58.01 213.79,57.01 213.79,53.6 IC1.10
N$100
  Top 0.25: C65.1 255.9,46.26 | 255.9,46.26 C46.1 | 255.9,46.26 257.15,45.01 R105.1 265.46,49.93 R106.2
N$104  (via drill 0.35)
  Top 0.25: R111.1 286.97,45.06 C50.2 284.45,39.01 244.79,39.01 v243.79,40.01
  Route15 0.25: v243.79,40.01 243.79,42.01 242.79,43.01 224.79,43.01 223.79,44.01 223.79,45.01 222.83,45.97 IC1.3
N$105
  Top 0.25: C66.1 277.3,46.25 C49.1 278.46,45.22 R110.1 286.98,50.47 R111.2
N$106
  Route2 0.25: IC14.7 176.71,56.09 177.79,55.01 186.19,55.01 IC11.6
N$107
  Top 0.25: IC11.8 178.89,55.01 168.65,55.01 IC14.11
N$108
  Bottom 0.25: LED6.A 203.44,21.2 R127.2
N$109
  Top 0.25: C53.2 308.83,41.29 308.83,45.08 R116.1
  Route2 0.25: C53.2 307.6,41.2 304.79,44.01 290.79,44.01 289.79,45.01 289.79,47.01 285.75,51.05 IC1.5
N$110
  Top 0.25: C67.1 C52.1 300.22,45.21 303.59,45.21 | R116.2 308.79,50.42 303.59,45.21 | 303.59,45.21 R115.1
N$111
  Bottom 0.25: LED5.A 190.74,20.64 R142.2
N$112
  Bottom 0.25: LED1.A 177.94,21.01 R128.2
N$113
  Top 0.25: T9.3 176.06,17.69 LED1.K
N$114  (via drill 0.35)
  Top 0.25: R121.1 241.41,24.12 C56.2 239.41,18.34 v227.29,18.34
  Route2 0.25: IC16.12 212.04,18.34 v227.29,18.34
N$115
  Top 0.25: R121.2 241.34,28.69 R120.1 233.22,24.19 C55.1 227.33,25.16 C64.1
N$116
  Top 0.25: T8.3 188.6,17.72 LED5.K
N$117
  Top 0.25: T7.3 201.3,19.2 LED6.K
N$119  (via drill 0.35)
  Top 0.25: R126.1 C59.2 239.69,39.01 v227.79,39.01
  Route2 0.25: v227.79,39.01 217.79,39.01 211.25,45.55 IC1.12
N$120
  Top 0.25: C58.1 228,46.08 C68.1 233.97,44.59 R125.1 241.74,49.79 R126.2
N$121
  Top 0.25: OK1.1 R130.2
N$122
  Top 0.25: OK1.4 R131.2
N$123
  Top 0.25: OK2.1 172.61,114.11 R68.2
N$124
  Top 0.25: OK2.4 180.23,109.56 R133.2
N$125
  Top 0.25: OK3.1 242.27,112.86 R134.2
N$126
  Top 0.25: OK3.4 249.89,108.49 R135.2
N$127
  Bottom 0.25: T7.2 197.9,22.05 R118.1
N$128
  Bottom 0.25: T8.2 185.12,22.07 R122.1
N$129
  Bottom 0.25: T9.2 172.76,22.21 R123.1
N$130
  Top 0.25: R144.2 161.44,42.72 IC14.13
  Bottom 0.25: IC14.13 171.79,43.87 171.79,40.01 174.79,37.01 197.79,37.01 R118.2
N$131
  Top 0.25: R145.2 157.14,40.36 164.79,48.01 164.79,57.01 166.41,58.63 IC14.9
  Bottom 0.25: R145.2 158.79,39.92 158.79,40.01 164.79,40.01 168.79,36.01 185.58,36.01 R122.2
N$132
  Route2 0.25: R146.2 164.79,49.73 164.79,54.01 166.87,56.09 IC14.10
  Route15 0.25: R123.2 174.74,37.06 172.79,39.01 172.79,50.49 IC14.10
N$142
  Route2 0.25: T10.2 162.5,49.3 R144.1
N$143
  Route2 0.25: T11.2 157.23,48.53 R145.1
N$144
  Route2 0.25: T12.2 153.27,55.25 R146.1
N$151  (via drill 0.35)
  Top 0.25: R113.2 194.02,43.42 IC11.2 | v206.79,68.01 210.79,68.01 211.79,67.01 231.77,67.01 IC21.1
  Route2 0.25: v206.79,62.01 v206.79,68.01
  Bottom 0.25: R113.2 202.17,44.39 203.79,46.01 206.79,46.01 v206.79,62.01
N$152  (via drill 0.35)
  Top 0.25: R149.2 193.31,51.04 IC11.5
  Route2 0.25: v202.79,62.01 202.79,67.01 205.79,70.01 v206.79,70.01
  Route15 0.25: v206.79,70.01 223.79,70.01 224.79,71.01 233.23,71.01 IC21.2
  Bottom 0.25: R149.2 202.37,52.59 202.79,53.01 v202.79,62.01
N$153  (via drill 0.35)
  Top 0.25: R151.2 190.37,52.01 180.97,52.01 IC11.10
  Route2 0.25: v201.79,62.01 201.79,67.01 205.79,71.01 225.51,71.01 IC21.14
  Bottom 0.25: R151.2 201.22,56.44 201.79,57.01 v201.79,62.01
N$154  (via drill 0.35)
  Top 0.25: R112.2 188.31,40.19 IC11.1
  Route2 0.25: v207.79,62.01 207.79,67.01 208.79,68.01 210.79,68.01 211.79,67.01 245.79,67.01 248.2,69.42 IC20.1
  Bottom 0.25: R112.2 201.97,40.19 203.79,42.01 207.79,42.01 v207.79,62.01
N$155  (via drill 0.35)
  Top 0.25: R117.2 194.8,48.5 IC11.4 | IC20.2 246.21,72.43 244.79,71.01 224.79,71.01 222.79,69.01 v206.79,69.01
  Route2 0.25: v203.79,62.01 203.79,67.01 205.79,69.01 v206.79,69.01
  Bottom 0.25: R117.2 202.37,48.59 203.79,50.01 v203.79,62.01
N$156  (via drill 0.35)
  Top 0.25: R150.2 189.61,55.01 181.43,55.01 IC11.9
  Route2 0.25: v200.79,62.01 200.79,67.01 205.79,72.01 223.44,72.01 225.01,73.58 237.22,73.58 240.58,70.22 IC20.14
  Bottom 0.25: R150.2 199.99,60.21 200.79,61.01 v200.79,62.01
N$157
  Top 0.25: J3.1 326.92,54.16 VR1.1 333.13,54.2 C18.2
N$158
  Top 1: R152.2 C20.1
N$163
  Bottom 1: R154.2 C23.1
N$164
  Bottom 1: R155.2 254.73,165.52 C27.1
NO  (via drill 0.35)
  Top 0.25: IC16.2 218.29,17.01 | 218.29,17.01 IC16.1 | C9.2 299.78,20.35 C61.2 295.14,20.35 293.38,22.11 | J9.2 293.34,27.6 293.34,22.15 293.38,22.11 | 293.38,22.11 289.28,18.01 248.79,18.01 246.79,16.01 219.29,16.01 218.29,17.01 | v146.79,15.01 62.79,15.01 55.79,22.01 55.79,67.42 R61.2
  Bottom 0.25: IC16.1 213.41,14.63 211.79,13.01 207.79,13.01 206.79,14.01 147.79,14.01 v146.79,15.01
NO1  (via drill 0.35)
  Top 0.25: IC16.7 IC16.6 | J11.2 271.36,27.33 | 271.36,27.33 271.36,21.89 273.02,20.24 C40.2 278.32,20.24 C62.2 | 271.36,27.33 271.36,34.44 267.79,38.01 v221.79,38.01
  Route2 0.25: IC16.7 221.79,33.37 v221.79,38.01 176.79,38.01 174.79,36.01 139.79,36.01 134.79,41.01 134.79,70.01 132.79,72.01 90.81,72.01 R99.2
NO2  (via drill 0.35)
  Top 0.25: IC16.8 IC16.9 139.11,27.33 135.79,24.01 135.79,20.01 132.79,17.01 64.79,17.01 59.66,22.14 R104.2 | C63.2 256.43,20.3 C43.2 249.27,22.4 249.27,27.22 249.42,27.38 | J13.2 249.42,27.38 | 249.42,27.38 249.42,32.38 244.79,37.01 217.79,37.01 214.47,33.69 v214.47,30.91
  Route2 0.25: v214.47,30.91 213.43,29.87 IC16.8
NO3  (via drill 0.35)
  Top 0.25: IC1.8 211.25,56.01 | 211.25,56.01 IC1.9 | C65.2 255.9,41.18 C46.2 250.62,41.18 248.79,43.01 248.79,48.04 | J15.2 248.79,48.04 | 248.79,48.04 248.79,51.01 241.79,58.01 213.25,58.01 211.25,56.01 | R109.2 50.79,62.99 50.79,71.01 54.79,75.01 134.79,75.01 142.79,67.01 v209.79,67.01
  Route15 0.25: v209.79,67.01 210.79,66.01 210.79,56.59 IC1.8
NO4  (via drill 0.35)
  Top 0.25: IC1.2 IC1.1 | C49.2 272.62,41.23 | 272.62,41.23 C66.2 | J17.2 270.79,48.85 270.79,43.01 272.57,41.23 272.62,41.23 | R114.2 81.67,73.01 134.79,73.01 142.79,65.01 v211.79,65.01
  Route2 0.25: C66.2 268.63,41.17 266.37,43.43 IC1.2
  Route15 0.25: v211.79,65.01 214.79,62.01 214.79,46.01 217.37,43.43 IC1.2
NO5  (via drill 0.35)
  Top 0.25: IC1.7 IC1.6 | C52.2 C67.2 | C67.2 | J19.2 296.74,52.71 292.41,48.38 | 292.41,48.38 292.41,42.37 293.42,41.36 C67.2 | 292.41,48.38 292.41,53.4 285.79,60.01 v223.79,60.01 | R119.2 50.57,50.01 51.79,50.01 51.79,71.01 54.79,74.01 134.79,74.01 142.79,66.01 v223.79,66.01
  Route2 0.25: v223.79,66.01 v223.79,60.01
  Bottom 0.25: v223.79,60.01 223.79,58.01 221.79,56.01 218.99,56.01 IC1.7
NO6  (via drill 0.35)
  Top 0.25: IC16.13 210.67,17.01 | 210.67,17.01 IC16.14 | C64.2 232.22,20.1 C55.2 | J21.2 225.39,27.53 225.39,22.02 C64.2 | C64.2 225.54,18.34 211.99,18.34 210.67,17.01 | R124.2 57.79,47.1 57.79,22.01 63.79,16.01 v147.79,16.01
  Bottom 0.25: IC16.14 149.17,14.63 v147.79,16.01
NO7  (via drill 0.35)
  Top 0.25: IC1.13 IC1.14 213.13,39.01 225.94,39.01 C58.2 | C58.2 232.44,41.04 C68.2 | J23.2 225.79,47.79 225.79,43.01 227.76,41.04 C58.2 | R129.2 121.89,39.01 124.79,39.01 125.79,38.01 v125.79,19.01
  Route15 0.25: v125.79,19.01 127.79,17.01 132.79,17.01 135.79,20.01 135.79,29.01 139.79,33.01 208.79,33.01 211.25,35.47 IC1.14
OC_PROTECTION_HIGH_REF  (via drill 0.35)
  Top 0.25: C35.1 167.62,73.49 VR10.2 165.38,68.85 J6.2 | IC20.5 246.79,81.46 246.79,83.72 | 246.79,83.72 IC20.7 | 246.79,83.72 245.66,82.59 IC20.9 236.16,87.01 v213.79,87.01
  Route2 0.25: v213.79,87.01 206.79,80.01 180.16,80.01 C35.1
OC_PROTECTION_LOW_REF
  Top 0.25: J7.2 195.52,75.7 VR11.2 198.59,72.69 202.79,72.69 C36.1 214.59,72.69 IC21.8 228.87,84.93 232.79,81.01 | IC21.4 232.79,78.97 232.79,81.01 | 232.79,81.01 234.17,82.39 IC21.6
PHASE_1
  Top 1: U4.6 111.36,148.74 C15.2 111.36,154.31 R37.2 108.11,157.7 D4.A Q1.S | Q2.D 129.99,166.52 D6.C
  pour Top: 105.96,177.34 105.96,187.26 145.79,187.26 150.51,182.54 150.51,178.05 148.75,178.05 142.54,184.26 133.29,184.26 132.1,183.07 132.1,177.65 131.46,177.01 128.66,177.01 127.9,177.77 127.9,183.32 127.21,184.01 111.04,184.01 110.35,183.32 110.35,177.71 109.65,177.01 106.29,177.01
PHASE_1_GRID
  Top 0.25: R5.1 404.79,167.99 404.79,168.01 395.79,168.01 | 395.79,168.01 394.46,166.68 R21.1 | X11.2 395.94,168.16 395.79,168.01
  pour Top: 328.91,178.13 328.91,182.26 396.79,182.26 399.29,179.76 399.29,171.51 398.54,170.76 344.54,170.76 338.29,177.01 330.03,177.01
PHASE_1_OUT
  pour Top: 146.04,193.26 154.79,193.26 156.29,191.76 156.29,180.01 154.54,178.26 151.79,178.26 151.36,178.69 151.36,184.69 148.54,187.51 147.54,187.51 146.04,189.01
PHASE_1_OUT_FILTERED
  pour Top: 328.16,177.43 328.16,185.63 329.29,186.76 332.54,186.76 333.29,187.51 333.29,193.01 332.04,194.26 325.29,194.26 323.29,192.26 323.29,179.76 325.62,177.43
PHASE_2
  Top 1: U6.6 180.33,147.91 C22.2 178.07,153.22 R51.2 D9.A 178.29,166.71 Q3.S | Q4.D 199.8,166.5 D10.C
  pour Top: 176.29,177.26 176.29,186.76 217.04,186.76 221.44,182.36 221.44,177.46 219.59,177.46 213.29,183.76 204.04,183.76 202.29,182.01 202.29,177.76 201.04,176.51 198.04,176.51 197.29,177.26 197.29,182.76 196.54,183.51 181.79,183.51 180.79,182.51 180.79,177.51 179.79,176.51 177.04,176.51
PHASE_2_GRID
  Top 0.25: R6.1 405.18,133.01 391.79,133.01 | R32.1 381.69,133.01 391.79,133.01 | X12.2 394.92,136.14 391.79,133.01
  pour Top: 343.07,142.3 343.07,145.79 343.29,146.01 345.54,146.01 346.04,146.51 397.04,146.51 399.54,144.01 399.54,135.76 398.79,135.01 355.29,135.01 349.29,141.01 344.36,141.01
PHASE_2_OUT_FILTERED  (via drill 0.35)
  other vias: 340.79,146.01 340.79,147.01 341.78,146.98 340.79,148.01 341.79,148.01 341.79,146.04
  pour Top: 339.54,148.26 339.54,141.31 342.36,141.31 342.36,149.01 340.29,149.01
  pour Bottom: 338.36,185.96 338.36,192.01 339.83,193.48 346.35,193.48 347.14,192.69 347.14,186.42 343.54,182.82 343.54,145.91 341.97,144.34 339.97,144.34 338.38,145.93 338.38,185.94
PHASE_3
  Top 1: 248.06,165.17 R57.2 248.06,151.5 C26.2 U7.6 | 248.06,165.17 D12.A | Q5.S 248.25,165.64 248.06,165.17 | Q6.D 269.84,165.45 D13.C
  pour Top: 293.79,177.76 293.79,182.83 289.86,186.76 247.54,186.76 245.97,185.19 245.97,177.08 247.29,175.76 250.29,175.76 252.04,177.51 252.04,181.76 252.79,182.51 267.29,182.51 267.79,182.01 267.79,178.01 268.79,177.01 272.04,177.01 272.04,183.01 289.29,183.01 290.64,181.66 290.64,177.76
PHASE_3_GRID
  Top 0.25: R22.1 404.04,98.01 392.13,98.01 | R33.1 381.49,98.01 392.13,98.01 | X13.2 392.13,98.01
  pour Top: 391.33,99.51 398.04,99.51 398.54,100.01 398.54,108.51 393.79,113.26 358.29,113.26 357.49,112.46 357.49,108.06 358.54,107.01 359.79,107.01 362.79,104.01 390.54,104.01 391.33,103.22
PHASE_3_OUT
  pour Top: 291.04,193.01 289.79,193.01 289.54,192.76 289.54,188.51 290.79,187.26 293.54,187.26 294.46,186.34 294.46,177.36 294.6,177.22 296.9,177.22 297.32,177.64 297.32,187.29 298.79,188.76 298.79,192.76 298.29,193.26 291.29,193.26
PHASE_3_OUT_FILTERED  (via drill 0.35)
  other vias: 356.04,116.26 355.04,116.26 354.04,116.26 354.04,115.26 355.04,115.26 356.04,115.26 356.04,114.26 355.04,114.26 354.04,114.26
  pour Top: 353.29,117.01 356.54,117.01 356.79,116.76 356.79,107.16 354.39,107.16 353.04,108.51 353.04,116.76
  pour Bottom: 353.09,186.59 353.09,192.64 354.56,194.11 361.08,194.11 361.87,193.32 361.87,187.05 357.51,182.69 357.51,112.46 357.12,112.07 354.18,112.07 353.11,113.14 353.11,113.11 353.09,113.09 353.11,186.57
PWM_A_NEG_OUTPUT
  Bottom 0.25: OK1.3 108.79,117.98 108.79,115.01 109.79,114.01 113.79,114.01 118.79,109.01 137.79,109.01 154.79,92.01 168.99,92.01 171.79,89.21 171.79,86.01 172.79,85.01 175.79,85.01 179.84,80.96 186.75,80.96 IC25.3
PWM_A_POS_OUTPUT
  Bottom 0.25: OK1.2 106.15,114.65 108.79,112.01 112.79,112.01 119.79,105.01 135.79,105.01 149.79,91.01 149.79,83.01 153.79,79.01 156.79,79.01 158.87,81.09 IC22.3
PWM_B_NEG_OUTPUT
  Route2 0.25: OK2.3 177.69,83.11 179.79,81.01 194.79,81.01 195.97,82.19 IC25.6
PWM_B_POS_OUTPUT
  Route2 0.25: OK2.2 175.15,87.37 174.79,87.01 167.79,87.01 166.49,85.71 IC22.6
PWM_C_NEG_OUTPUT
  Top 0.25: OK3.3 247.35,106.57 234.79,94.01 233.79,94.01 202.34,94.01 IC25.8
PWM_C_POS_OUTPUT  (via drill 0.35)
  Top 0.25: OK3.2 244.81,110.03 230.79,96.01 v171.79,96.01
  Route2 0.25: v171.79,96.01 171.79,92.74 IC22.8
TIM1_CH1  (via drill 0.35)
  Top 0.25: J1.23 132.22,49.01 135.79,49.01 136.79,50.01 136.79,63.01 v139.79,66.01
  Route2 0.25: v139.79,66.01 142.79,69.01 142.79,75.01 150.14,82.36 IC22.1
TIM1_CH1N  (via drill 0.35)
  Top 0.25: J1.30 127.69,56.11 126.79,57.01 v126.79,70.01
  Route15 0.25: v126.79,70.01 126.79,76.01 127.79,77.01 177.72,77.01 IC25.1
TIM1_CH2  (via drill 0.35)
  Top 0.25: J1.21 131.76,46.01 136.79,46.01 138.79,48.01 138.79,62.01 139.79,63.01 v146.79,63.01
  Route2 0.25: v146.79,63.01 161.41,77.63 IC22.4
TIM1_CH2N  (via drill 0.35)
  Top 0.25: J1.28 127.23,53.57 124.79,56.01 v124.79,70.01
  Route15 0.25: v124.79,70.01 124.79,77.01 133.79,86.01 187.79,86.01 190.89,82.91 IC25.4
TIM1_CH3  (via drill 0.35)
  Top 0.25: v138.27,67.49 131.97,61.19 J1.33
  Route2 0.25: v138.27,67.49 140.79,70.01 140.79,76.01 150.79,86.01 163.79,86.01 166.49,88.71 IC22.9
TIM1_CH3N  (via drill 0.35)
  Top 0.25: J1.26 129.14,51.01 126.79,51.01 122.79,55.01 v122.79,70.01
  Route15 0.25: v122.79,70.01 122.79,80.01 141.79,99.01 189.79,99.01 195.97,92.83 IC25.9
TYT
  pour Top: 217.04,192.51 225.79,192.51 227.29,191.01 227.29,179.26 225.54,177.51 222.79,177.51 222.24,178.81 222.18,184.12 219.54,186.76 218.54,186.76 217.04,188.26
VOLTAGE_MEAS_DC_LINK  (via drill 0.35)
  Top 0.25: J21.1 229.67,34.35 R120.2 238.5,36.01 241.79,36.01 243.79,34.01 243.79,19.01 v245.79,17.01 | R47.1 340.2,37.66 J12.1 338.09,37.71 336.79,39.01 317.79,39.01 v316.79,38.01
  Route2 0.25: v316.79,38.01 311.79,33.01 311.79,20.01 314.62,17.18 IC7.14
  Bottom 0.25: v245.79,17.01 319.32,17.01 IC7.14
VOLTAGE_MEAS_PHASE_1_TO_2
  Top 0.25: J9.1 297.69,34.41 R14.2 306.21,36.01 313.79,36.01 315.79,34.01 315.79,20.01 317.34,18.46 325.83,18.46 IC7.1 328.96,17.18 330.79,19.01 330.79,24.01 337.79,31.01 386.97,31.01 J4.1 393.66,37.71 R44.1
VOLTAGE_MEAS_PHASE_1_TO_3  (via drill 0.35)
  Top 0.25: J11.1 282.56,34.25 R62.2 285.32,37.01 314.79,37.01 317.79,34.01 v317.79,31.01 | R45.1 J8.1
  Route2 0.25: v317.79,31.01 325.7,31.01 326.75,32.05 IC7.7 329.7,35.01 373.63,35.01 J8.1
VOLTAGE_MEAS_PHASE_2_TO_3  (via drill 0.35)
  Top 0.25: R100.2 254.03,34.52 J13.1 | R46.1 358.99,37.66 J10.1 355.18,34.01 v323.79,34.01
  Route2 0.25: v323.79,34.01 322.2,32.42 IC7.8
  Bottom 0.25: R100.2 264.66,38.01 315.79,38.01 319.49,34.31 IC7.8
